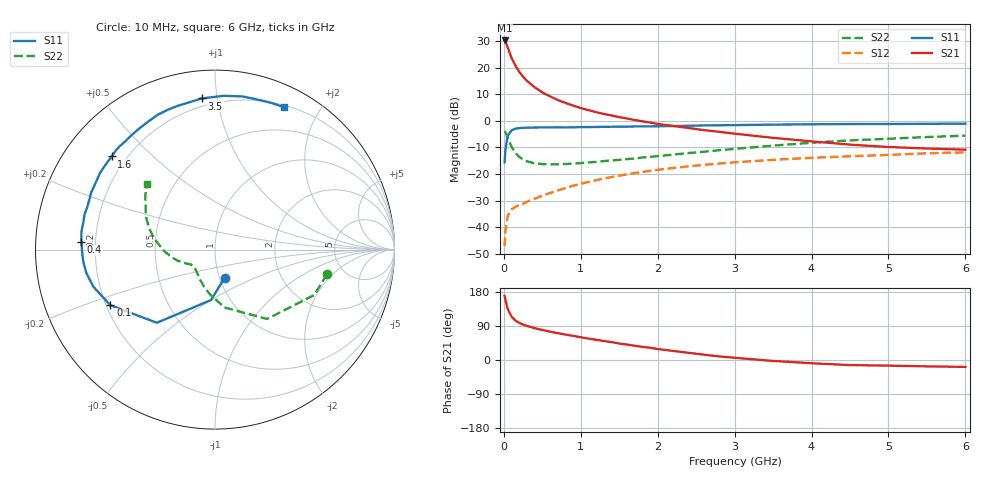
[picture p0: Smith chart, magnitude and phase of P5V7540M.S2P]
! SIEMENS Small Signal Semiconductors
! BFP183
! Si NPN RF Bipolar Junction Transistor in SOT143
! VCE = 0.75 V  IC = 40 mA
! Common Emitter S-Parameters:  March  1996
# GHz  S  MA  R  50
!  f  S11  S21  S12  S22
! GHz  MAG  ANG  MAG  ANG  MAG  ANG  MAG  ANG
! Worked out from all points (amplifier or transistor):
!   36 points, 10 MHz to 6 GHz, reference 50 ohm
!   highest |S21| = 30.2 dB at 10 MHz (marker M1)
!   |S21| within 3 dB of that: start of sweep to 55.23 MHz
!   unconditionally stable (mu >= 1): start of sweep to 23.96 MHz; 181.5 MHz to end of sweep
!   at 250 MHz: K = 1.22, MAG = 21.0 dB, |S12| = -31.2 dB
!   at 1.4 GHz: K = 1.89, MAG = 6.1 dB, |S12| = -21.1 dB
!   at 6 GHz: K = 1.54, MAG = -3.8 dB, |S12| = -11.9 dB
!   S11 on the Smith chart (normalised r, x): 10 MHz: 1.06, -0.34; 100 MHz: 0.22, -0.24; 400 MHz: 0.15, +0.03; 1.6 GHz: 0.15, +0.38; 3.5 GHz: 0.15, +0.91; 6 GHz: 0.22, +1.57
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0.01  0.1659 -71.1  32.25 169.2  0.0044 70.0  0.6385 -12.4
0.02  0.2819 -94.5  30.84 159.0  0.0084 66.3  0.6087 -24.5
0.05  0.5207 -128.5  23.94 134.9  0.0162 51.6  0.4833 -53.1
0.1  0.6604 -152.0  15.21 114.6  0.0216 39.4  0.3264 -80.8
0.15  0.7088 -163.1  10.85 104.3  0.0241 37.8  0.2496 -96.8
0.2  0.7279 -169.5  8.317 98.0  0.026 39.8  0.2101 -108.0
0.25  0.7364 -174.3  6.734 93.4  0.0276 41.4  0.1872 -116.2
0.3  0.7392 -177.6  5.653 89.9  0.03 43.3  0.1727 -122.2
0.4  0.7459 176.9  4.255 84.0  0.0342 47.8  0.1587 -130.9
0.5  0.7505 172.5  3.404 79.3  0.0389 50.4  0.1532 -136.9
0.6  0.7492 168.4  2.876 74.8  0.0439 52.9  0.152 -140.9
0.7  0.7528 164.8  2.454 70.9  0.0489 54.6  0.1517 -143.4
0.9  0.753 158.7  1.93 63.7  0.0601 55.9  0.1569 -147.3
1.1  0.7608 152.3  1.58 56.5  0.0712 55.8  0.1645 -150.7
1.3  0.7699 146.3  1.342 50.1  0.0821 54.9  0.1746 -153.3
1.6  0.7745 137.9  1.103 40.8  0.0985 53.0  0.19 -157.0
2.2  0.7948 122.6  0.799 23.9  0.1293 46.9  0.2312 -167.0
2.8  0.8227 108.4  0.619 9.4  0.157 39.6  0.2797 -177.6
3.5  0.8454 94.9  0.477 -2.5  0.1843 31.6  0.3411 170.3
4.5  0.8671 79.8  0.356 -13.5  0.2151 20.3  0.428 154.2
5.5  0.8756 69.0  0.301 -16.8  0.2445 10.6  0.4941 141.8
6  0.8809 64.3  0.286 -18.2  0.2546 5.3  0.5242 136.0
